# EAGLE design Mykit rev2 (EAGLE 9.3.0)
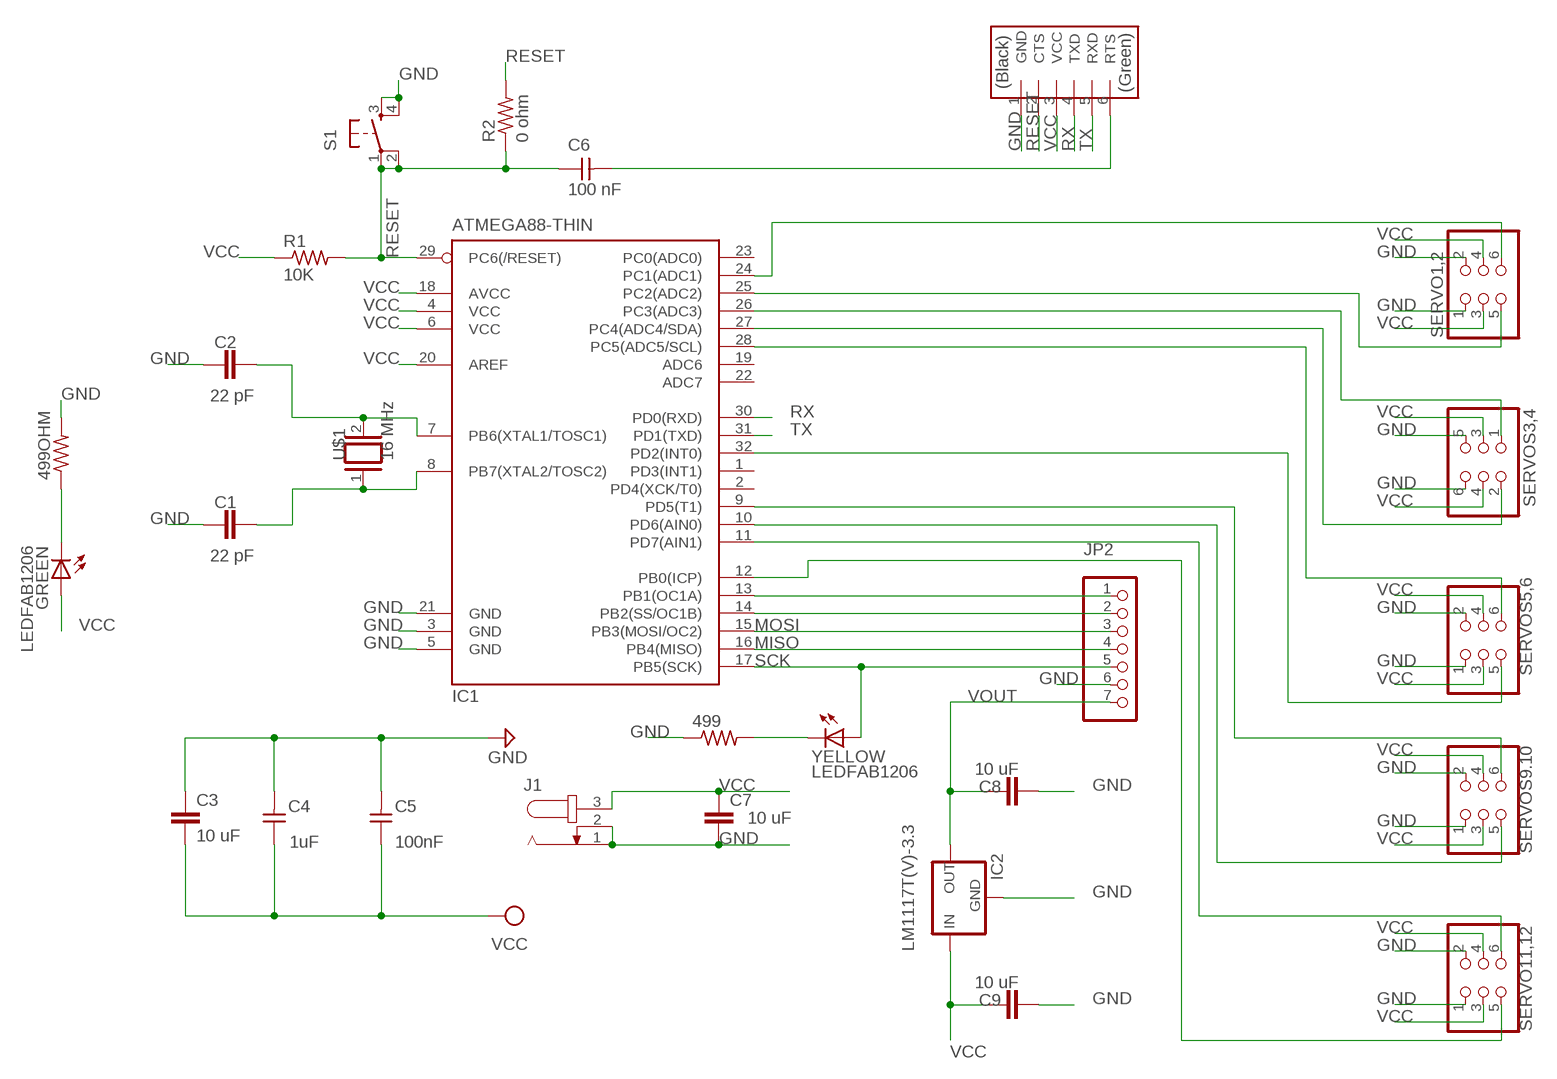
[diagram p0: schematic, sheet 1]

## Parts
499  RES-US1206FAB  [R1206FAB]
499OHM  RES-US1206FAB  [R1206FAB]
C1  22 pF  C-EUC0603  [C0603]
C2  22 pF  C-EUC0603  [C0603]
C3  10 uF  C-EUC1808  [C1808]
C4  1uF  CAP-UNPOLARIZEDFAB  [C1206FAB]
C5  100nF  CAP-UNPOLARIZEDFAB  [C1206FAB]
C6  100 nF  CAP-UNPOLARIZEDFAB  [C1206FAB]
C7  10 uF  C-EUC1808  [C1808]
C8  10 uF  C-EUC1808  [C1808]
C9  10 uF  C-EUC1808  [C1808]
GREEN  LEDFAB1206  [LED1206FAB]
IC1  ATMEGA88-THIN  [TQFP32-08THIN]
IC2  LM1117T(V)-3.3  [TO220V]
J1  JACK-PLUG1  [SPC4078]
JP2  PINHD-1X07_2.54-SMD  [1X07SMD]
R1  10K  RES-US1206FAB  [R1206FAB]
R2  0 ohm  RES-US1206FAB  [R1206FAB]
S1  6MM_SWITCH6MM_SWITCH  [6MM_SWITCH]
SERVO1,2  PINHD-2X3-SMD  [2X03SMD]
SERVO11,12  PINHD-2X3-SMD  [2X03SMD]
SERVOS3,4  PINHD-2X3-SMD  [2X03SMD]
SERVOS5,6  PINHD-2X3-SMD  [2X03SMD]
SERVOS9.10  PINHD-2X3-SMD  [2X03SMD]
U$1  16 MHz  XTAL/S  [QS]
U$3  FTDI-SMD-HEADER  [1X06SMD]
YELLOW  LEDFAB1206  [LED1206FAB]

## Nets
GND: 499.1 499OHM.2 C1.1 C2.1 C3.1 C4.2 C5.2 C7.2 C8.2 C9.2 IC1.3(GND) IC1.5(GND) IC1.21(GND) IC2.1(GND) J1.1 J1.2 JP2.6 S1.3(S) S1.4(S1) SERVO1,2.1 SERVO1,2.2 SERVO11,12.1 SERVO11,12.2 SERVOS3,4.5 SERVOS3,4.6 SERVOS5,6.1 SERVOS5,6.2 SERVOS9.10.1 SERVOS9.10.2 U$3.1(GND)
MISO: IC1.16(PB4(MISO)) JP2.4
MOSI: IC1.15(PB3(MOSI/OC2)) JP2.3
N$1: C2.2 IC1.7(PB6(XTAL1/TOSC1)) U$1.2
N$2: C1.2 IC1.8(PB7(XTAL2/TOSC2)) U$1.1
N$3: IC1.13(PB1(OC1A)) JP2.1
N$4: IC1.14(PB2(SS/OC1B)) JP2.2
N$5: IC1.27(PC4(ADC4/SDA)) SERVOS3,4.2
N$6: IC1.26(PC3(ADC3)) SERVOS3,4.1
N$7: 499OHM.1 GREEN.2(C)
N$9: 499.2 YELLOW.2(C)
N$11: C6.2 U$3.6(RTS)
N$14: IC1.9(PD5(T1)) SERVOS9.10.6
N$15: IC1.10(PD6(AIN0)) SERVOS9.10.5
N$16: IC1.11(PD7(AIN1)) SERVO11,12.6
N$17: IC1.12(PB0(ICP)) SERVO11,12.5
N$21: IC1.28(PC5(ADC5/SCL)) SERVOS5,6.6
N$23: IC1.24(PC1(ADC1)) SERVO1,2.6
N$24: IC1.25(PC2(ADC2)) SERVO1,2.5
N$25: IC1.32(PD2(INT0)) SERVOS5,6.5
RESET: C6.1 IC1.29(PC6(/RESET)) R1.2 R2.1 R2.2 S1.1(P) S1.2(P1) U$3.2(CTS)
RX: IC1.30(PD0(RXD)) U$3.4(TXD)
SCK: IC1.17(PB5(SCK)) JP2.5 YELLOW.1(A)
TX: IC1.31(PD1(TXD)) U$3.5(RXD)
VCC: C3.2 C4.1 C5.1 C7.1 C9.1 GREEN.1(A) IC1.4(VCC) IC1.6(VCC) IC1.18(AVCC) IC1.20(AREF) IC2.3(IN) J1.3 R1.1 SERVO1,2.3 SERVO1,2.4 SERVO11,12.3 SERVO11,12.4 SERVOS3,4.3 SERVOS3,4.4 SERVOS5,6.3 SERVOS5,6.4 SERVOS9.10.3 SERVOS9.10.4 U$3.3(VCC)
VOUT: C8.1 IC2.2(OUT) JP2.7
Unconnected: IC1.1(PD3(INT1)) IC1.2(PD4(XCK/T0)) IC1.19(ADC6) IC1.22(ADC7) IC1.23(PC0(ADC0))

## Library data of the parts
499 499OHM R1 R2 = eagle_fab:RES-US: Resistor (US Symbol)
C1-C3 C7-C9 = rcl:C-EU: CAPACITOR, European symbol; SPICEPREFIX: C
C4-C6 = eagle_fab:CAP-UNPOLARIZED
GREEN YELLOW = eagle_fab:LED: LED
IC1 = eagle_fab:ATMEGA88-THIN
IC2 = lm1117_10:LM1117?-*: 800mA Low-Dropout Linear Regulator Source: http://www.ti.com/lit/ds/symlink/lm1117-n.pdf; MF: Texas Instruments; MPN: LM1117T-3.3; OC_FARNELL: 1469056; OC_NEWARK: 13B5347
J1 = con-jack:JACK-PLUG: DC POWER JACK Power Jack, DC, Right Angle, Through Hole, Rated 5A at 16VDC, PC Terminals Distributor: Farnell (www.Farnell.de) Drawing: 84N1161.pdf / 84N1162.pdf Manufacturer: SPC Technology (www.spctechnology.com) Type: SPC4077 / SPC 4078; OC_FARNELL: unknown; OC_NEWARK: unknown
JP2 = pinhead-2:PINHD-1X07: PIN HEADER
S1 = eagle_fab:6MM_SWITCH: OMRON SWITCH
SERVO1,2 SERVO11,12 SERVOS3,4 SERVOS5,6 SERVOS9.10 = eagle_fab:PINHD-2X3-SMD: PIN HEADER
U$1 = special:XTAL/S: CRYSTAL
U$3 = eagle_fab:FTDI-SMD-HEADER

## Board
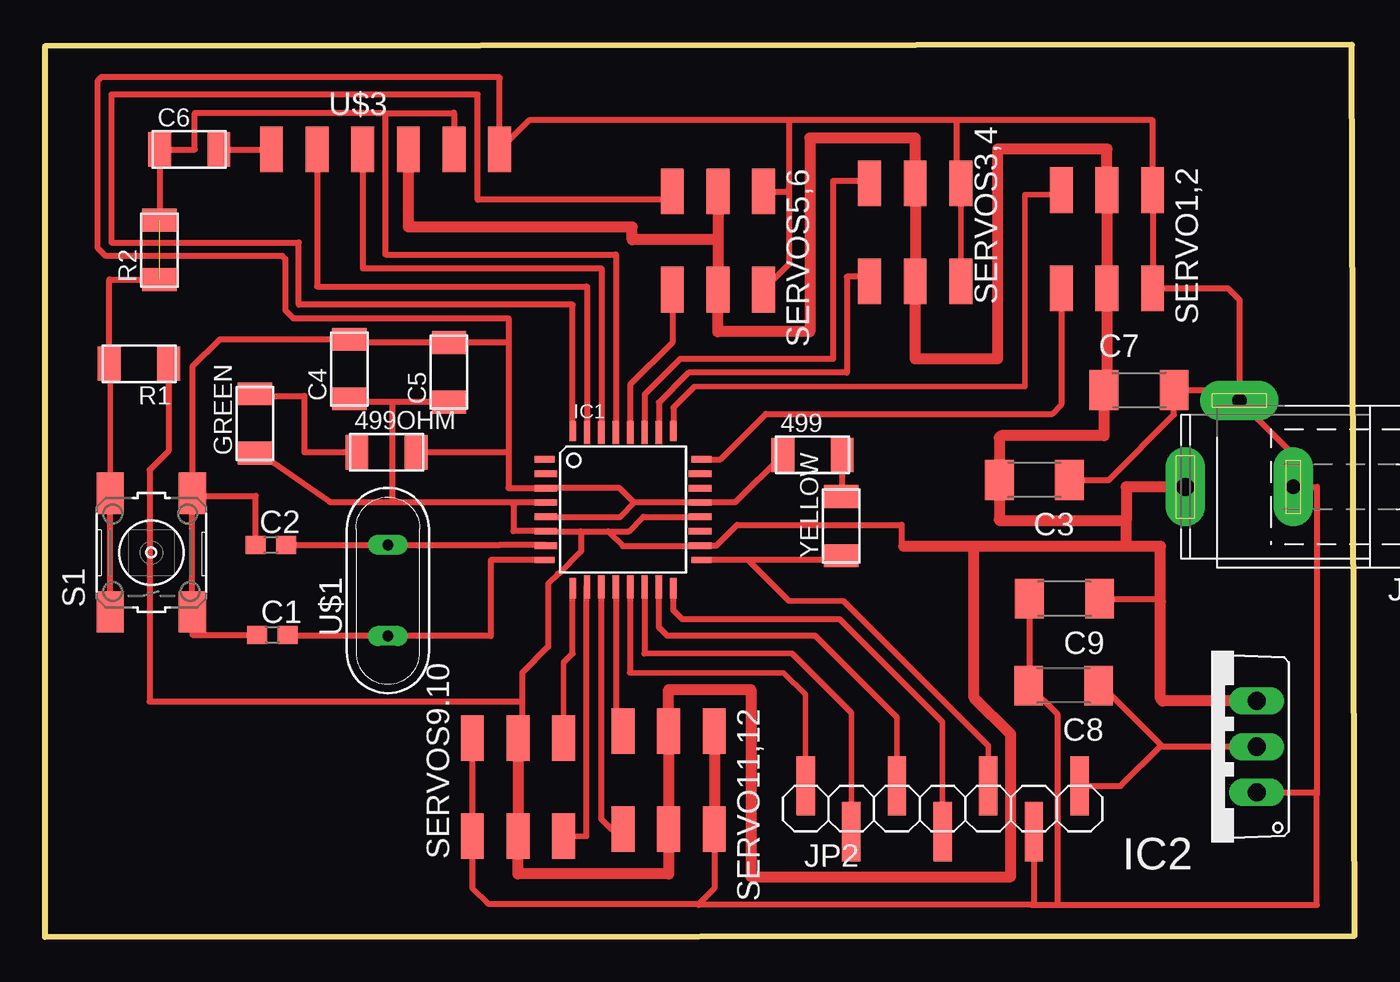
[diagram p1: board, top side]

Size 72.85 x 49.63 mm. Coordinates in mm from the lower left corner, seen from the top.
Outline: 0,0 72.85,0.08 72.7,49.63 0,49.56 0,0
Copper layers (1*16): Top 0.035mm / dielectric 1.5mm / Bottom 0.035mm
Design rules "fabmodule": minimum track width 10mil, minimum drill 0.4mm, track to track 0.42mm, track to pad 0.42mm, pad to pad 0.42mm, via to via 0.42mm, smd to smd 0.42mm, copper to edge 40mil, drill to drill 0.8mm, minimum pad ring 10mil, minimum via ring 8mil, stop-mask expansion 4mil, vias tented up to drill 0mil, thermal gap 10mil

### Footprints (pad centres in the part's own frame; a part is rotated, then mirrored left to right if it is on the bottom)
R1206FAB = smd 1.27 x 1.905: 1 -1.651,0; 2 1.651,0
C0603 = smd 1.1 x 1: 1 -0.85,0; 2 0.85,0
C1808 = smd 1.6 x 2.2: 1 -1.95,0; 2 1.95,0
C1206FAB = smd 1.27 x 1.905: 1 -1.651,0; 2 1.651,0
LED1206FAB = smd 1.27 x 1.905: 1 -1.651,0; 2 1.651,0
TQFP32-08THIN = smd 1.118 x 0.356: 1 -4.369,2.8; 8 -4.369,-2.8; 17 4.369,-2.8; 24 4.369,2.8 | smd 1.27 x 0.356: 2 -4.293,2; 3 -4.293,1.2; 4 -4.293,0.4; 5 -4.293,-0.4; 6 -4.293,-1.2; 7 -4.293,-2; 18 4.293,-2; 19 4.293,-1.2; 20 4.293,-0.4; 21 4.293,0.4; 22 4.293,1.2; 23 4.293,2 | smd 0.356 x 1.118: 9 -2.8,-4.369; 16 2.8,-4.369; 25 2.8,4.369; 32 -2.8,4.369 | smd 0.356 x 1.27: 10 -2,-4.293; 14 1.2,-4.293; 15 2,-4.293; 26 2,4.293; 27 1.2,4.293; 31 -2,4.293 | smd 0.35 x 1.27: 11 -1.2,-4.293; 12 -0.4,-4.293; 13 0.4,-4.293; 28 0.4,4.293; 29 -0.4,4.293; 30 -1.2,4.293
TO220V = drill 1.016 long: 1 -2.54,-2.54; 2 0,-2.54; 3 2.54,-2.54
SPC4078 = drill 0.8 pad 2.184 long: 1 -3,0; 2 0,-4.8 | drill 1 pad 2.184 long: 3 3,0
1X07SMD = smd 1.016 x 3.302: 1 -1.27,1.27; 2 1.27,-1.27; 3 3.81,1.27; 4 6.35,-1.27; 5 8.89,1.27; 6 11.43,-1.27; 7 13.97,1.27
6MM_SWITCH = smd 2.286 x 1.524: 1 -3.302,2.286; 2 3.302,2.286; 3 -3.302,-2.286; 4 3.302,-2.286
2X03SMD = smd 2.54 x 1.27: 1 -2.54,2.54; 2 2.92,2.54; 3 -2.54,0; 4 2.92,0; 5 -2.54,-2.54; 6 2.92,-2.54
QS = drill 0.61 long: 1 -2.54,0; 2 2.54,0
1X06SMD = smd 2.54 x 1.27: 1 0,6.35; 2 0,3.81; 3 0,1.27; 4 0,-1.27; 5 0,-3.81; 6 0,-6.35

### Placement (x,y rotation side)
499  42.7,26.82 0 top
499OHM  19,26.97 0 top
C1  12.65,16.81 0 top
C2  12.57,21.82 0 top
C3  55.04,25.43 180 top
C4  16.94,31.6 90 top
C5  22.48,31.42 90 top
C6  8.03,43.82 0 top
C7  60.86,30.43 0 top
C8  56.67,14 180 top
C9  56.72,18.82 180 top
GREEN  11.68,28.58 90 top
IC1  32.16,23.77 0 top
IC2  64.87,10.59 90 top
J1  66.45,25.04 180 top
JP2  43.59,7.14 0 top
R1  5.23,31.9 180 top
R2  6.38,38.23 90 top
S1  5.92,21.39 90 top
SERVO1,2  59.08,39.01 270 top
SERVO11,12  34.7,8.92 270 top
SERVOS3,4  48.41,39.01 90 top
SERVOS5,6  37.44,38.94 270 top
SERVOS9.10  26.31,8.15 90 top
U$1  19.08,19.28 90 top
U$3  18.95,43.82 270 top
YELLOW  44.3,22.86 90 top

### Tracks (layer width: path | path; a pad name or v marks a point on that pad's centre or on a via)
GND
  Top 0.254: 17.12,33.07 C4.2
  Top 0.305: SERVOS3,4.6 50.95,41.3 SERVOS3,4.5
  Top 0.33: 41.4,45.44 41.4,41.61 | 41.4,41.61 41.28,41.48 SERVOS5,6.1 | 41.4,41.61 41.4,37.44 SERVOS5,6.2 | SERVOS9.10.2 SERVOS9.10.1 23.77,2.72 24.64,1.85 36.37,1.85 | SERVO11,12.2 37.24,2.72 36.37,1.85 | 54.89,1.78 36.37,1.78 36.37,1.85 | C1.1 8.2,16.81 S1.3 S1.4 | 50.7,45.44 61.62,45.44 SERVO1,2.1 SERVO1,2.2 65.81,36.09 66.45,35.46 J1.2 | 50.7,45.44 50.7,41.55 50.95,41.3 | 50.7,45.44 41.4,45.44 | 41.4,45.44 26.92,45.44 U$3.1 25.3,47.79 25.24,47.85 21.58,47.85 21.57,47.85 3.15,47.85 2.95,47.65 2.95,38.32 3.39,37.88 13.21,37.88 13.37,37.72 13.37,34.87 13.81,34.43 25.78,34.43 25.78,33.07 | IC1.21 32.77,24.17 31.97,24.97 IC1.3 25.8,24.97 25.78,24.99 25.78,26.97 | IC1.21 32.81,24.17 31.98,23.34 27.9,23.34 IC1.5 | S1.4 8.2,24.54 11.72,24.54 C2.1 | J1.2 69.45,26.84 J1.1 70.76,25.04 70.76,7.92 | 25.78,33.07 C5.2 17.12,33.07 | 25.78,33.07 25.78,26.97 | J1.2 65.86,30.43 C7.2 62.81,29.06 59.18,25.43 C3.1 | C4.2 9.72,33.25 8.2,31.73 S1.4 | 70.76,7.92 70.76,1.78 56.34,1.78 | 54.84,18.75 C9.2 54.77,13.94 C8.2 56.34,12.38 56.34,1.78 | IC2.1 70.64,8.05 70.76,7.92 | JP2.6 55.02,1.91 54.89,1.78 | 499.1 38.4,24.17 IC1.21 | 499OHM.2 25.78,26.97 | 54.89,1.78 56.34,1.78
  Top 0.61: SERVO11,12.1 SERVO11,12.2
MISO
  Top 0.305: JP2.4 49.94,11.96 44.22,17.68
  Top 0.33: IC1.16 34.96,18.18 35.46,17.68 44.22,17.68
MOSI
  Top 0.305: JP2.3 47.4,12.22 42.85,16.76
  Top 0.33: 42.85,16.76 34.62,16.76 34.16,17.23 IC1.15
N$1
  Top 0.33: IC1.7 27.86,21.81 25.31,21.81 25.31,21.82 U$1.2 C2.2
N$2
  Top 0.33: IC1.8 24.79,20.97 24.79,16.74 U$1.1 13.58,16.74 C1.2
N$3
  Top 0.305: JP2.1 42.32,13.49 41.1,14.71 32.54,14.71 | IC1.13 32.54,19.46
  Top 0.33: 32.54,19.46 32.54,14.71
N$4
  Top 0.305: JP2.2 44.86,12.47 41.55,15.77 33.35,15.77 | IC1.14
  Top 0.33: IC1.14 33.35,15.77
N$5
  Top 0.33: IC1.27 33.36,30.18 35.33,32.16 43.84,32.16 43.84,42.06 45.87,42.06 SERVOS3,4.2
N$6
  Top 0.33: SERVOS3,4.1 45.62,36.73 44.6,36.73 44.6,31.39 35.81,31.39 34.16,29.74 IC1.26
N$7
  Top 0.33: GREEN.2 11.81,30.1 14.43,30.1 14.43,26.97 499OHM.1
N$9
  Top 0.33: 499.2 44.35,24.56 YELLOW.2
N$11
  Top 0.33: C6.2 U$3.6
N$14
  Top 0.305: SERVOS9.10.6 28.85,15.27 29.36,15.77 | IC1.9
  Top 0.33: 29.36,15.77 IC1.9
N$15
  Top 0.305: SERVOS9.10.5 30.12,5.61 | 30.12,19.45 IC1.10
  Top 0.33: 30.12,5.61 30.12,19.45
N$16
  Top 0.305: SERVO11,12.6 31.52,6 30.94,6.58 | IC1.11 30.96,19.29 30.94,19.27
  Top 0.33: 30.94,19.27 30.94,6.58
N$17
  Top 0.305: SERVO11,12.5 31.78,11.84 | IC1.12 31.78,19.46
  Top 0.33: 31.78,19.46 31.78,11.84
N$21
  Top 0.33: SERVOS5,6.6 34.9,33.07 32.56,30.73 IC1.28
N$23
  Top 0.33: SERVO1,2.6 56.54,29.62 56.03,29.11 40.11,29.11 37.57,26.57 IC1.24
N$24
  Top 0.305: SERVO1,2.5 56.29,41.3 54.51,41.3 54.51,30.63 36.14,30.63 34.96,29.44
  Top 0.33: 34.96,29.44 IC1.25
N$25
  Top 0.33: SERVOS5,6.5 34.44,41.02 24.08,41.02 24.08,46.88 3.7,46.88 3.7,38.63 14.12,38.63 14.12,35.18 29.36,35.18 IC1.32
RESET  (1 unrouted)
  Top 0.305: S1.2 3.63,31.85 R1.2
  Top 0.33: 18.95,45.85 18.95,37.97 31.76,37.97 IC1.29 | S1.1 S1.2 | 18.95,45.85 8.33,45.85 8.33,43.82 C6.1 R2.2 | R1.2 3.58,36.58 R2.1 | 18.95,45.85 22.71,45.85 22.73,45.87 22.76,45.85 U$3.2
RX
  Top 0.33: U$3.4 17.68,37.21 30.96,37.21 IC1.30
SCK
  Top 0.305: JP2.5 52.48,10.64 44.43,18.69 41.4,18.69 39.12,20.97
  Top 0.33: IC1.17 39.12,20.97 44.06,20.97 YELLOW.1
TX
  Top 0.33: U$3.5 15.14,36.2 30.12,36.2 30.16,36.16 IC1.31
VCC
  Top 0.33: 29.82,22.57 IC1.6 26.06,22.58 26.06,24.03 26.21,24.17 | 29.82,22.57 31.32,22.57 | 31.32,22.57 32.16,21.74 36.42,21.74 IC1.18 37.34,21.77 38.51,22.94 47.65,22.94 47.65,21.87 47.78,21.74 | 31.32,22.57 32.48,22.57 33.28,23.37 IC1.20 | IC1.4 26.21,24.17 | 29.82,22.57 29.82,21.44 28.59,20.21 28.54,20.21 27.99,19.66 27.99,16.15 26.54,14.71 26.54,13.11 | 26.54,13.11 26.54,11.3 SERVOS9.10.4 | 26.54,13.11 5.82,13.11 5.82,25.98 6.88,27.05 R1.1 | C4.1 17.12,29.77 19.23,29.77 | 26.21,24.17 19.3,24.17 | 19.3,24.17 15.87,24.17 15.82,24.23 11.91,26.92 GREEN.1 | 59.06,36.07 SERVO1,2.4 | 62.18,13.13 62.05,13.26 | C9.1 61.9,18.82 62.05,18.67 | C5.1 19.23,29.77 | 19.23,29.77 19.3,29.69 19.3,24.17
  Top 0.61: SERVOS5,6.3 37.44,38.79 | 37.44,38.79 SERVOS5,6.4 37.44,33.68 42.55,33.68 42.55,44.45 48.41,44.45 SERVOS3,4.4 SERVOS3,4.3 48.41,32.16 52.98,32.16 52.98,43.84 59.08,43.84 SERVO1,2.3 SERVO1,2.4 | SERVOS9.10.4 SERVOS9.10.3 26.31,3.51 34.7,3.51 SERVO11,12.4 SERVO11,12.3 34.7,13.77 39.27,13.77 39.27,3.35 53.72,3.35 53.72,11.28 51.69,13.31 51.69,21.74 | 37.44,38.79 32.66,38.79 32.66,39.5 20.22,39.5 U$3.3 | J1.3 60.15,25.04 60.15,23.16 | 60.15,21.74 60.15,23.16 | 47.78,21.74 51.69,21.74 | 51.69,21.74 60.15,21.74 | 60.15,21.74 62.05,21.74 62.05,18.67 62.05,13.26 | 59.06,36.07 59.06,30.58 C7.1 58.91,27.89 53.19,27.89 53.09,27.79 C3.2 53.09,23.22 53.14,23.16 60.15,23.16 | IC2.3 62.18,13.13
VOUT
  Top 0.33: 62.1,10.67 58.77,14 C8.1 | 62.1,10.67 59.84,8.41 JP2.7 | IC2.2 62.17,10.59 62.1,10.67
